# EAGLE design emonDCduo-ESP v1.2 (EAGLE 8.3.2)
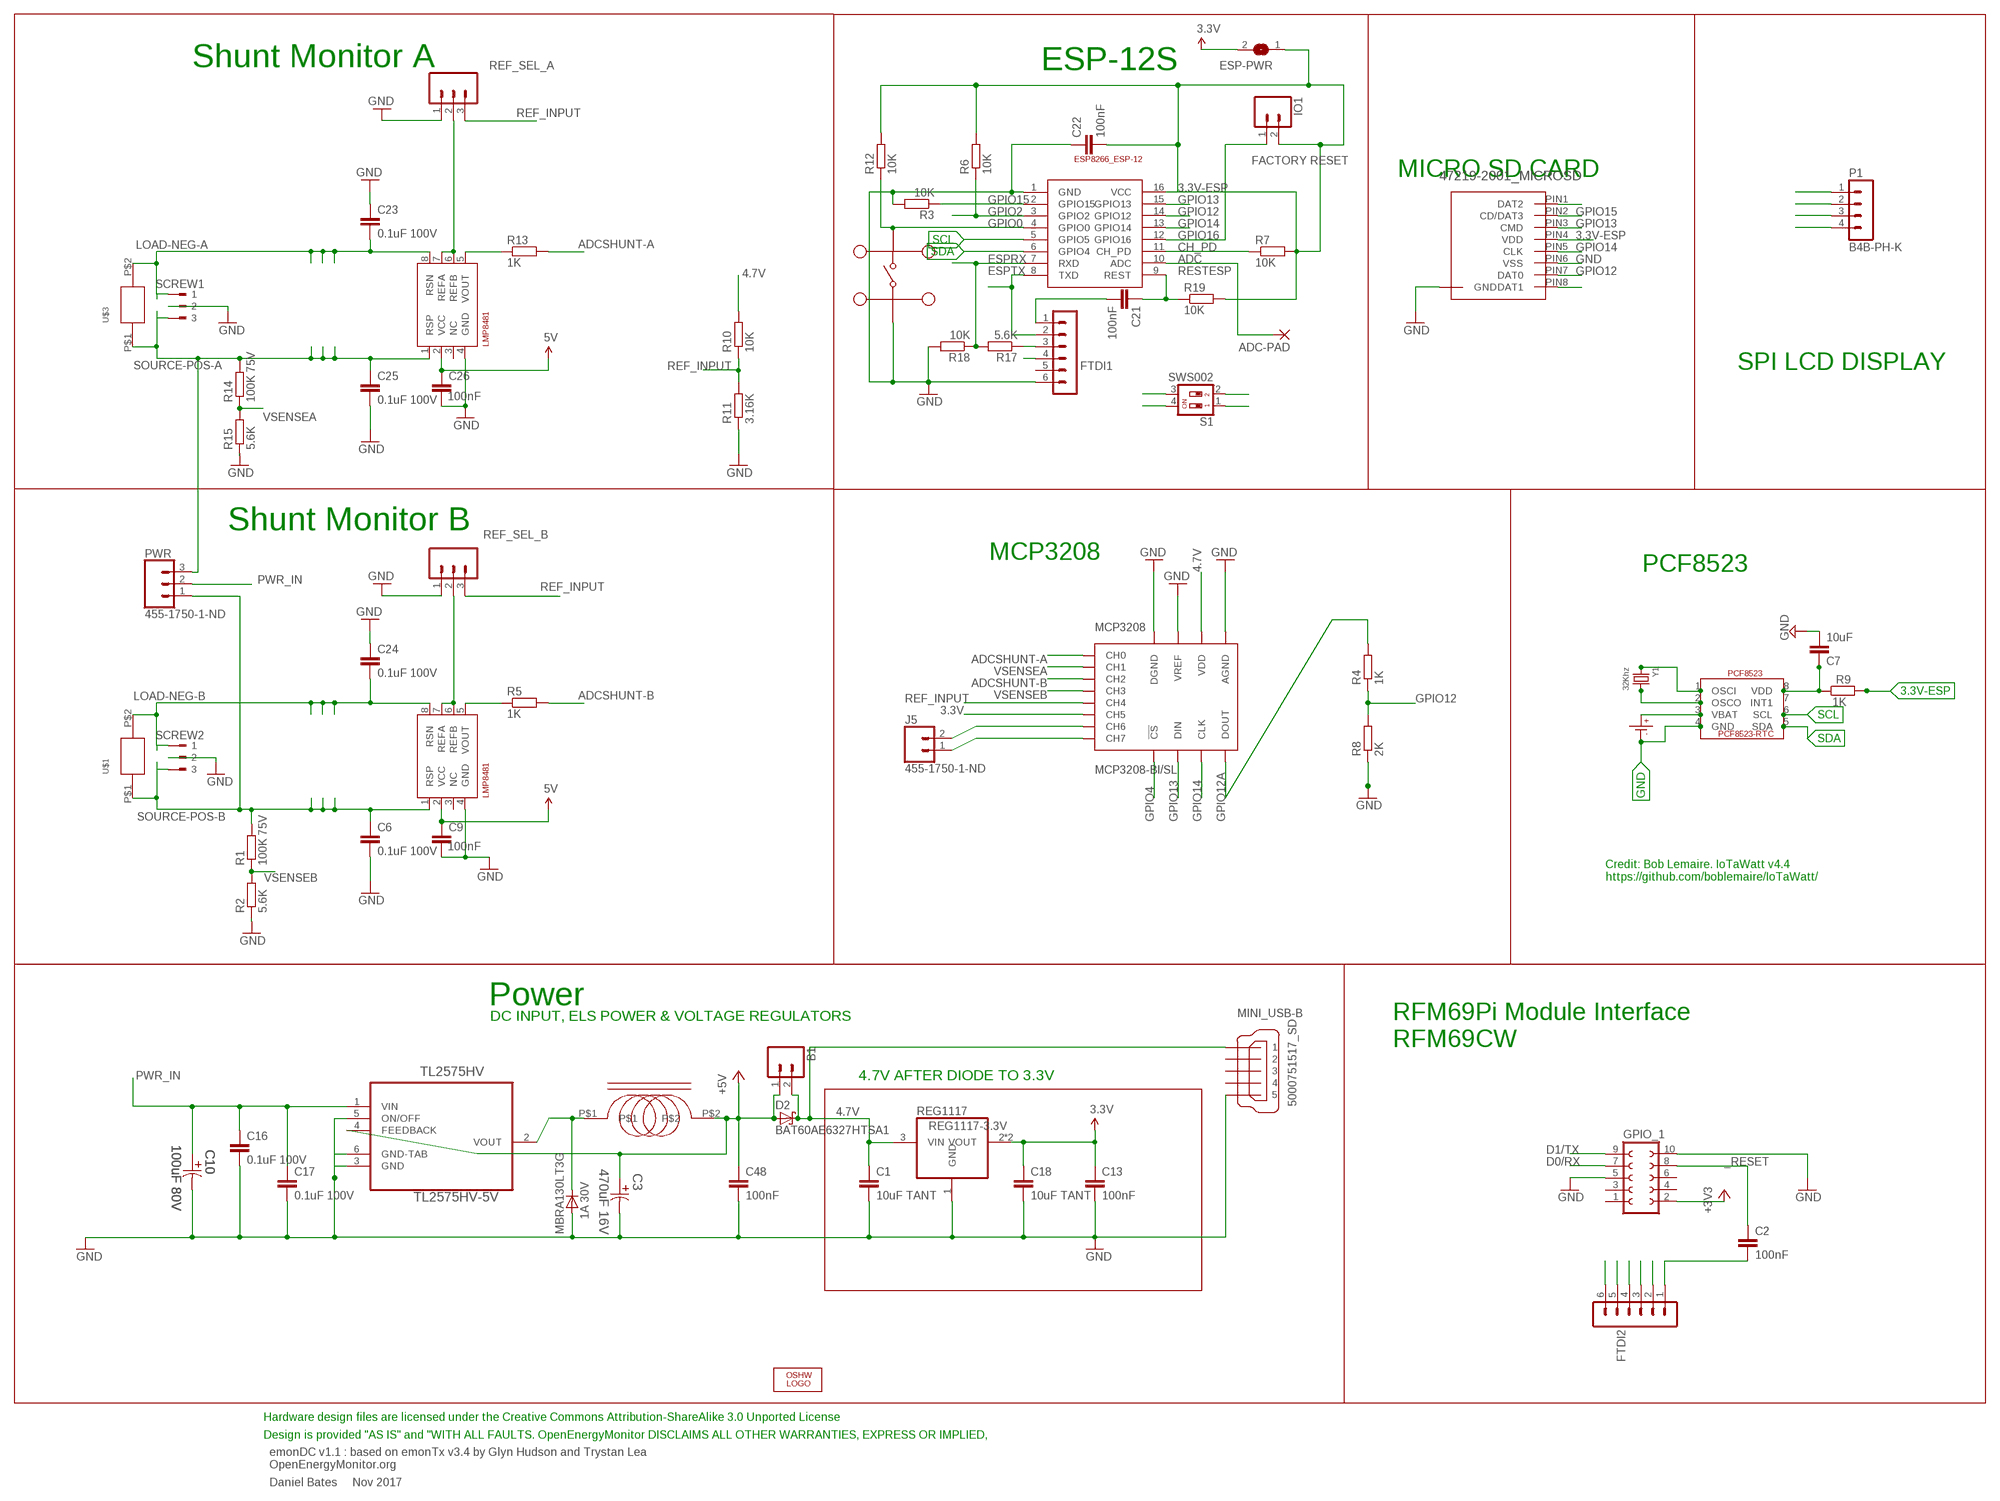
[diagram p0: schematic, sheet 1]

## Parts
ADC-PAD  2,15/1,0  [2,15/1,0]
B1  M02PTH  [1X02]
C1  10uF TANT  C-EUC0603  [C0603]
C2  100nF  C-EUC0603  [C0603]
C3  470uF 16V  EEE-FK1C471P-CASE-F  [CAPAE830X1050N]
C6  0.1uF 100V  C-EUC0603  [C0603]
C7  10uF  C-EUC0603  [C0603]
C9  100nF  C-EUC0603  [C0603]
C10  100uF 80V  EEV-FK1K101Q-CASE-H13  [CAPAE1350X1400N]
C13  100nF  C-EUC0603  [C0603]
C16  0.1uF 100V  C-EUC0603  [C0603]
C17  0.1uF 100V  C-EUC0603  [C0603]
C18  10uF TANT  C-EUC0603  [C0603]
C21  100nF  C-EUC0603  [C0603]
C22  100nF  C-EUC0603  [C0603]
C23  0.1uF 100V  C-EUC0603  [C0603]
C24  0.1uF 100V  C-EUC0603  [C0603]
C25  0.1uF 100V  C-EUC0603  [C0603]
C26  100nF  C-EUC0603  [C0603]
C48  100nF  C-EUC0603  [C0603]
CR1220  CR1220SMD  [CR1220SMD]
D1  MBRA130LT3G  [DO-214]
D2  BAT60AE6327HTSA1  BAT60J  [SOD323_ST]
ESP-12  ESP8266_ESP-12  [ESP8266-ESP12]
ESP-PWR  SJ  [SJ]
FTDI1  FTDI  MA06-1  [MA06-1]
FTDI2  FTDI  MA06-1  [MA06-1]
GPIO_1  FE05-2  [FE05-2]
I1  330uH  SRR0603-331KL  [SRR0603-331KL]
IO1  M02PTH  [1X02]
J5  455-1750-1-ND  CONN_02  [1X02]
LOGO1  OSHW_LOGO_6MILX0200-NT  [OSHW_6X200_NOTEXT]
MC2  MC32882  [SWITCH_TACT_MULTICOMP]
MCP3208  MCP3208-BI/SL  [SOIC16]
MINI_USB-B  5000751517_SD  [5000751517_SD]
P1  B4B-PH-K  [B4B-PH-K]
PCF8523  PCF8523_RTC  [SOIC_8]
PWR  455-1750-1-ND  CONN_03  [1X03]
R1  100K 75V  R-EU_R0603  [R0603]
R2  5.6K  R-EU_R0603  [R0603]
R3  10K  R-EU_R0603  [R0603]
R4  1K  R-EU_R0603  [R0603]
R5  1K  R-EU_R0603  [R0603]
R6  10K  R-EU_R0603  [R0603]
R7  10K  R-EU_R0603  [R0603]
R8  2K  R-EU_R0603  [R0603]
R9  1K  R-EU_R0603  [R0603]
R10  10K  R-EU_0309/12  [0309/12]
R11  3.16K  R-EU_0309/12  [0309/12]
R12  10K  R-EU_R0603  [R0603]
R13  1K  R-EU_R0603  [R0603]
R14  100K 75V  R-EU_R0603  [R0603]
R15  5.6K  R-EU_R0603  [R0603]
R17  5.6K  R-EU_R0603  [R0603]
R18  10K  R-EU_R0603  [R0603]
R19  10K  R-EU_R0603  [R0603]
REF_SEL_A  455-1750-1-ND  CONN_03  [1X03]
REF_SEL_B  455-1750-1-ND  CONN_03  [1X03]
REG1117  REG1117-3.3V  REG1117-VOUT4  [SOT223]
S1  SWS002  [SMS-002]
SCREW1  180-3  [180-3]
SCREW2  180-3  [180-3]
SHUNTMON-A  LMP8481  LMP8481-H  [S-PDSO-G08]
SHUNTMON-B  LMP8481  LMP8481-H  [S-PDSO-G08]
TL2575HV  TL2575HV-5V  TL2575HV-05IKTTR  [TO-263]
U$1  EBW_SERIES_15.2MM  [EBW_SERIES_15.2MM]
U$3  EBW_SERIES_15.2MM  [EBW_SERIES_15.2MM]
U$4  47219-2001_MICROSD  [47219-2001_MICROSD]
Y1  32Khz  CRYSTAL8X3.8SMT  [CRYSTAL_8X3.8]

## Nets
3.3V: C13.1 C18.1 ESP-PWR.2 GPIO_1.2 MCP3208.6(CH5) P1.3 REG1117.2(VOUT) REG1117.4(VOUT) ; supply symbol labelled +3V3
3.3V-ESP: C22.2 ESP-12.16(VCC) ESP-PWR.1 IO1.2 R6.2 R7.2 R9.2 R12.2 R19.2 U$4.PIN4(VDD)
4.7V [power]: B1.2 C1.1 C9.1 C26.1 D2.C FTDI1.4 FTDI2.4 MCP3208.16(VDD) MINI_USB-B.VBUS R10.2 REG1117.3(VIN) SHUNTMON-A.2(VCC) SHUNTMON-B.2(VCC) ; supply symbol labelled 5V
+5V: B1.1 C3.1 C48.1 D2.A I1.P$2 TL2575HV.4(FEEDBACK)
_RESET: C2.1 GPIO_1.8
ADC: ADC-PAD.1(P) ESP-12.10(ADC)
ADCSHUNT-A: MCP3208.1(CH0) R13.2
ADCSHUNT-B: MCP3208.3(CH2) R5.2
CH6: J5.2 MCP3208.7(CH6)
CH7: J5.1 MCP3208.8(CH7)
CH_PD: ESP-12.11(CH_PD) R7.1
D0/RX: FTDI2.2 GPIO_1.7 S1.2
D1/TX: FTDI2.3 GPIO_1.9 S1.1
ESPRX: ESP-12.7(RXD) R17.2 R18.1 S1.4
ESPTX: ESP-12.8(TXD) FTDI1.2 S1.3
GND [thin_power]: C1.2 C3.2 C6.2 C7.2 C9.2 C10.2 C13.2 C16.2 C17.2 C18.2 C22.1 C23.1 C24.1 C25.2 C26.2 C48.2 CR1220.P-(P$-) D1.P$2(A) ESP-12.1(GND) FTDI1.6 FTDI2.6 GPIO_1.5 GPIO_1.10 MC2.P$1 MC2.P$2 MCP3208.9(DGND) MCP3208.14(AGND) MCP3208.15(VREF) MINI_USB-B.GND1 MINI_USB-B.GND2 MINI_USB-B.GND3 P1.4 PCF8523.4(GND) R2.1 R3.2 R8.1 R11.1 R15.1 R18.2 REF_SEL_A.1 REF_SEL_B.1 REG1117.1(GND) SCREW1.2 SCREW2.2 SHUNTMON-A.4(GND) SHUNTMON-B.4(GND) TL2575HV.3(GND) TL2575HV.5(ON/OFF) TL2575HV.6(GND-TAB) U$4.P$1(GND) U$4.P$2(GND) U$4.P$3(GND) U$4.P$4(GND) U$4.PIN6(VSS)
GPIO0: ESP-12.4(GPIO0) MC2.P$3 MC2.P$4 R12.1
GPIO2: ESP-12.3(GPIO2) R6.1
GPIO4: MCP3208.10(!CS)
GPIO12: ESP-12.14(GPIO12) R4.1 R8.2 U$4.PIN7(DAT0)
GPIO12A: MCP3208.12(DOUT) R4.2
GPIO13: ESP-12.15(GPIO13) MCP3208.11(DIN) U$4.PIN3(CMD)
GPIO14: ESP-12.13(GPIO14) MCP3208.13(CLK) U$4.PIN5(CLK)
GPIO15 [thin_power]: ESP-12.2(GPIO15) R3.1 U$4.PIN2(CD/DAT3)
GPIO16: ESP-12.12(GPIO16) IO1.1
IND: D1.P$1(C) I1.P$1 TL2575HV.2(VOUT)
LOAD-NEG-A: C23.2 SCREW1.1 SHUNTMON-A.8(RSN) U$3.P$2
LOAD-NEG-B: C24.2 SCREW2.1 SHUNTMON-B.8(RSN) U$1.P$2
N$4: R13.1 SHUNTMON-A.5(VOUT)
N$6: R5.1 SHUNTMON-B.5(VOUT)
N$7: U$4.PIN1(DAT2)
N$10: C7.1 PCF8523.8(VDD) R9.1
N$20: FTDI2.5
N$30: C21.2 FTDI1.1
N$32: U$4.PIN8(DAT1)
N$36: FTDI1.3 R17.1
N$43: CR1220.P+(P$+) PCF8523.3(VBAT)
N$44: PCF8523.2(OSCO) Y1.P$4
N$45: PCF8523.1(OSCI) Y1.P$1
N$301: C2.2 FTDI2.1
PWR_IN: C10.1 C16.1 C17.1 PWR.2 TL2575HV.1(VIN)
REF_A_INPUT: REF_SEL_A.2 SHUNTMON-A.6(REFB) SHUNTMON-A.7(REFA)
REF_B_INPUT [thin_power]: REF_SEL_B.2 SHUNTMON-B.6(REFB) SHUNTMON-B.7(REFA)
REF_INPUT: MCP3208.5(CH4) R10.1 R11.2 REF_SEL_A.3 REF_SEL_B.3
RESTESP: C21.1 ESP-12.9(REST) R19.1
SCL: ESP-12.5(GPIO5) P1.2 PCF8523.6(SCL)
SDA: ESP-12.6(GPIO4) P1.1 PCF8523.5(SDA)
SOURCE-POS-A: C25.1 PWR.3 R14.2 SCREW1.3 SHUNTMON-A.1(RSP) U$3.P$1
SOURCE-POS-B: C6.1 PWR.1 R1.2 SCREW2.3 SHUNTMON-B.1(RSP) U$1.P$1
VSENSEA: MCP3208.2(CH1) R14.1 R15.2
VSENSEB: MCP3208.4(CH3) R1.1 R2.2
Unconnected: FTDI1.5 GPIO_1.1 GPIO_1.3 GPIO_1.4 GPIO_1.6 MINI_USB-B.D+ MINI_USB-B.D- MINI_USB-B.ID PCF8523.7(INT1) SHUNTMON-A.3(NC) SHUNTMON-B.3(NC)

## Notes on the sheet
- Shunt Monitor A | ESP-12S
- FACTORY RESET
- MICRO SD CARD
- SPI LCD DISPLAY
- Shunt Monitor B
- MCP3208
- PCF8523
- Credit: Bob Lemaire. IoTaWatt v4.4
  https://github.com/boblemaire/IoTaWatt/
- Power
- DC INPUT, ELS POWER & VOLTAGE REGULATORS
- RFM69Pi Module Interface
  RFM69CW
- 4.7V AFTER DIODE TO 3.3V
- Hardware design files are licensed under the Creative Commons Attribution-ShareAlike 3.0 Unported License
- Design is provided "AS IS" and "WITH ALL FAULTS. OpenEnergyMonitor DISCLAIMS ALL OTHER WARRANTIES, EXPRESS OR IMPLIED,
- emonDC v1.1 : based on emonTx v3.4 by Glyn Hudson and Trystan Lea
  OpenEnergyMonitor.org
- Daniel Bates     Nov 2017

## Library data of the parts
ADC-PAD = wirepad:2,15/1,0: THROUGH-HOLE PAD
B1 IO1 = SparkFun:M02: Header 2
C1 C2 C7 C13 C16-C18 C21 C22 C48 = rcl:C-EU: CAPACITOR, European symbol
C3 = Panasonic-EEEFK_EEEFP:EEE-: Aluminum Electrolytic Capacitors,Surface Mount Type; MPN: EEE-FK1C471P; OC_FARNELL: 9695710; OC_NEWARK: 96K9385; PACKAGE: CASE-F; SUPPLIER: PANASONIC; TOLERANCE: ±20 %; VALUE: 470UF; VOLTAGERATING: 16V
C6 C9 C23-C26 = rcl:C-EU: CAPACITOR, European symbol; MPN: C1608X7S2A104K080AB
C10 = Panasonic-EEE-EEV-EEF-ECQ:EEV-: Aluminum Electrolytic Capacitors,Surface Mount Type; MPN: EEVFK1K101Q; OC_FARNELL: 9696113; OC_NEWARK: 96K9484; SUPPLIER: PANASONIC; TOLERANCE: ±20 %; VALUE: 100UF; VOLTAGERATING: 80V
CR1220 = IotaWatt_parts:CR1220SMD: CR1220 Battery SMD
D1 = CASE 403D Diode:MBRA130LT3G: Fast switching diode; MF: ON SEMICONDUCTOR; MPN: MBRA130LT3G; OC_FARNELL: 9555978
D2 = diode:BAT60J: Schottky barrier diode
ESP-12 = ESP8266-ESP12:ESP8266_ESP-12
ESP-PWR = jumper:SJ: SMD solder JUMPER
FTDI1 FTDI2 = JeeLabs:MA06-1: PIN HEADER
GPIO_1 = con-lsta:FE05-2: FEMALE HEADER; OC_FARNELL: unknown; OC_NEWARK: unknown
I1 = SRR0603-331KL:SRR0603-331KL: SRR0603-331KL; INDUCTANCE: 330uH; MF: BOURNS; MPN: SRR0603-331KL; OC_FARNELL: 2333890
J5 = SparkFun-Connectors:CONN_02: Multi connection point. Often used as Generic Header-pin footprint for 0.1 inch spaced/style header connections
LOGO1 = ohw-logo:OSHW_LOGO_6MIL; OC_FARNELL: unknown
MC2 = multicomp tact switch:MC32882
MCP3208 = MCP3208:MCP3208
MINI_USB-B = 5000751517_sd:5000751517_SD
P1 = jst-ph:B4B-PH-K: HEADER
PCF8523 = IotaWatt_parts:PCF8523_RTC: PCF8523-RTC SOIC-8
PWR = SparkFun-Connectors:CONN_03: Multi connection point. Often used as Generic Header-pin footprint for 0.1 inch spaced/style header connections On any of the 0.1 inch spaced packages, you can populate with these: Break Away Headers - Straight (PRT-00116) Break Away Male Headers - Right Angle (PRT-00553) Female Headers (PRT-00115)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; PROD_ID: XXX-00000
R1 R14 = rcl:R-EU_: RESISTOR, European symbol; MPN: MCWR06X1003FTL
R2 R4 R8 R15 = rcl:R-EU_: RESISTOR, European symbol; MPN: MCWR06X5901FTL
R3 R5-R7 R9-R13 R17-R19 = rcl:R-EU_: RESISTOR, European symbol
REF_SEL_A REF_SEL_B = SparkFun-Connectors:CONN_03: Multi connection point. Often used as Generic Header-pin footprint for 0.1 inch spaced/style header connections On any of the 0.1 inch spaced packages, you can populate with these: Break Away Headers - Straight (PRT-00116) Break Away Male Headers - Right Angle (PRT-00553) Female Headers (PRT-00115)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; MF: MULTICOMP; MPN: 2212S-02SG-85; OC_FARNELL: 1593458; PROD_ID: XXX-00000
REG1117 = burr-brown:REG1117-VOUT4: 800mA and 1A Low Dropout (LDO) Positive Regulator 1.8V, 2.5V, 2.85V, 3.3V, 5V, and Adj; MF: TEXAS INSTRUMENTS; MPN: REG1117; OC_FARNELL: 1097566; OC_NEWARK: 14P6981
S1 = smd-special:SWS002: SMD Dip Switch 2 pol.
SCREW1 SCREW2 = con-weidmueller-sl35:180-3: WEIDMUELLER CLAMP CONNECTOR; OC_FARNELL: unknown; OC_NEWARK: unknown
SHUNTMON-A = lmp8481b:LMP8481: LMP8481MM-H/NOPB 100V/V; MF: TEXAS INSTRUMENTS; MPN: LMP8481MME-S/NOPB; OC_FARNELL: 2322044
SHUNTMON-B = lmp8481b:LMP8481: LMP8481MM-H/NOPB 100V/V; MF: TEXAS INSTRUMENTS; MPN: LMP8481MME-H/NOPB; OC_FARNELL: 2322044
TL2575HV = TL2575HV:TL2575HV; MF: TEXAS INSTRUMENTS; MPN: LM2575HVS-15/NOPB; OC_FARNELL: 2492609
U$1 U$3 = EBW series shunt:EBW_SERIES_15.2MM
U$4 = MOLEX 47219-2001:47219-2001_MICROSD
Y1 = microbuilder:CRYSTAL: Crystals

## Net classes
2 thin_power: width 0.254 mm

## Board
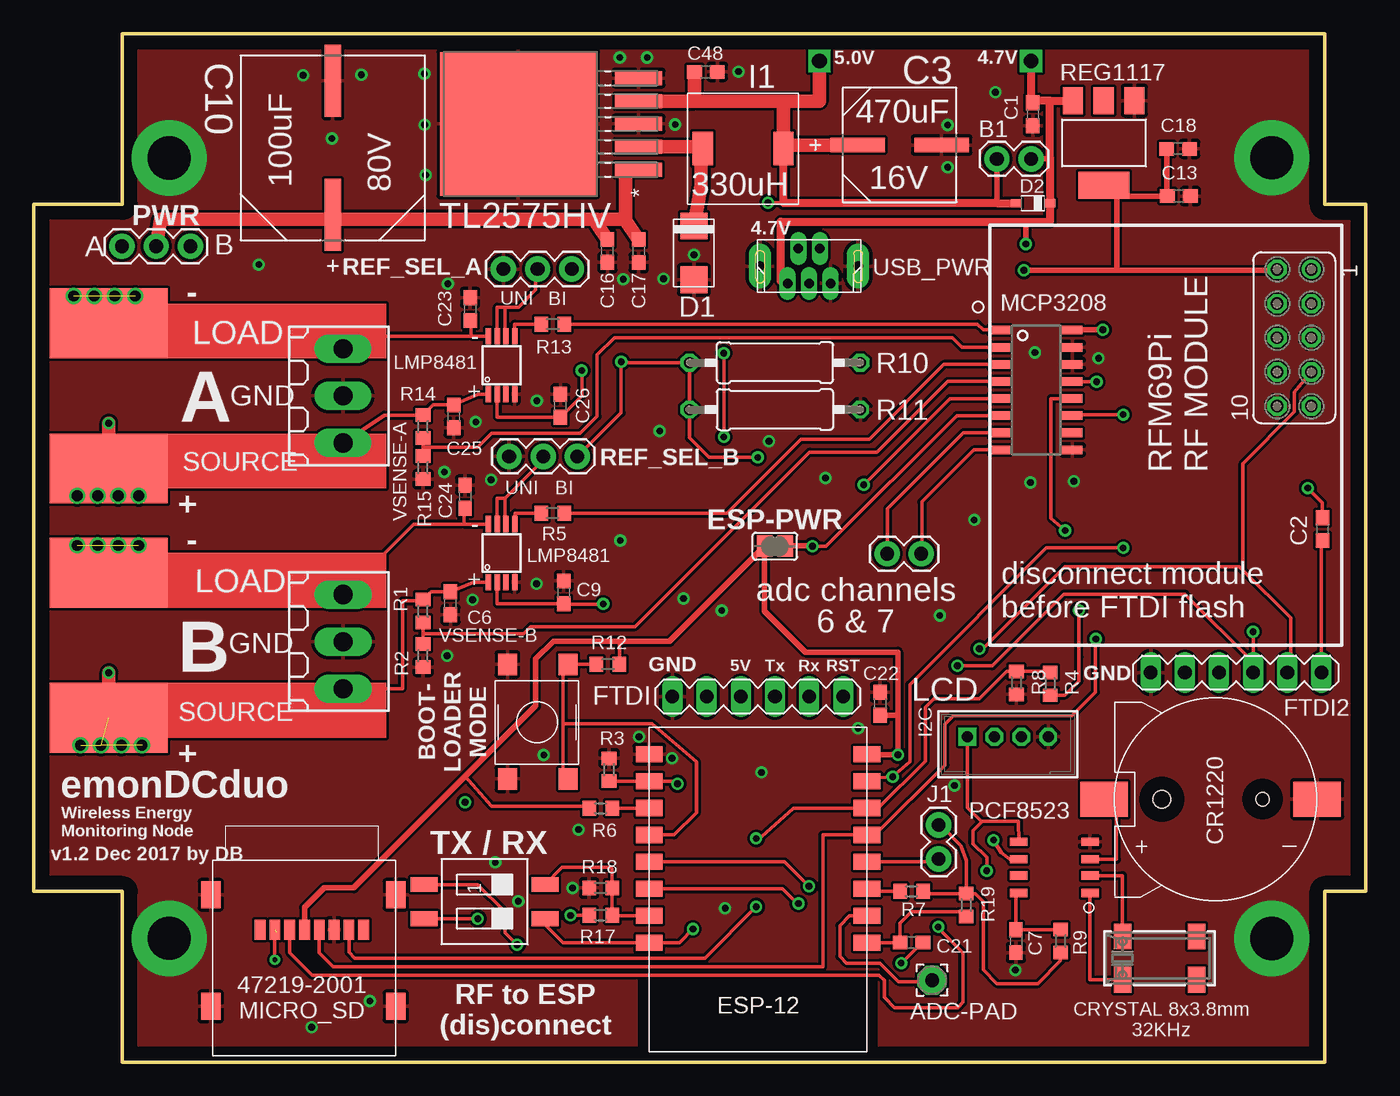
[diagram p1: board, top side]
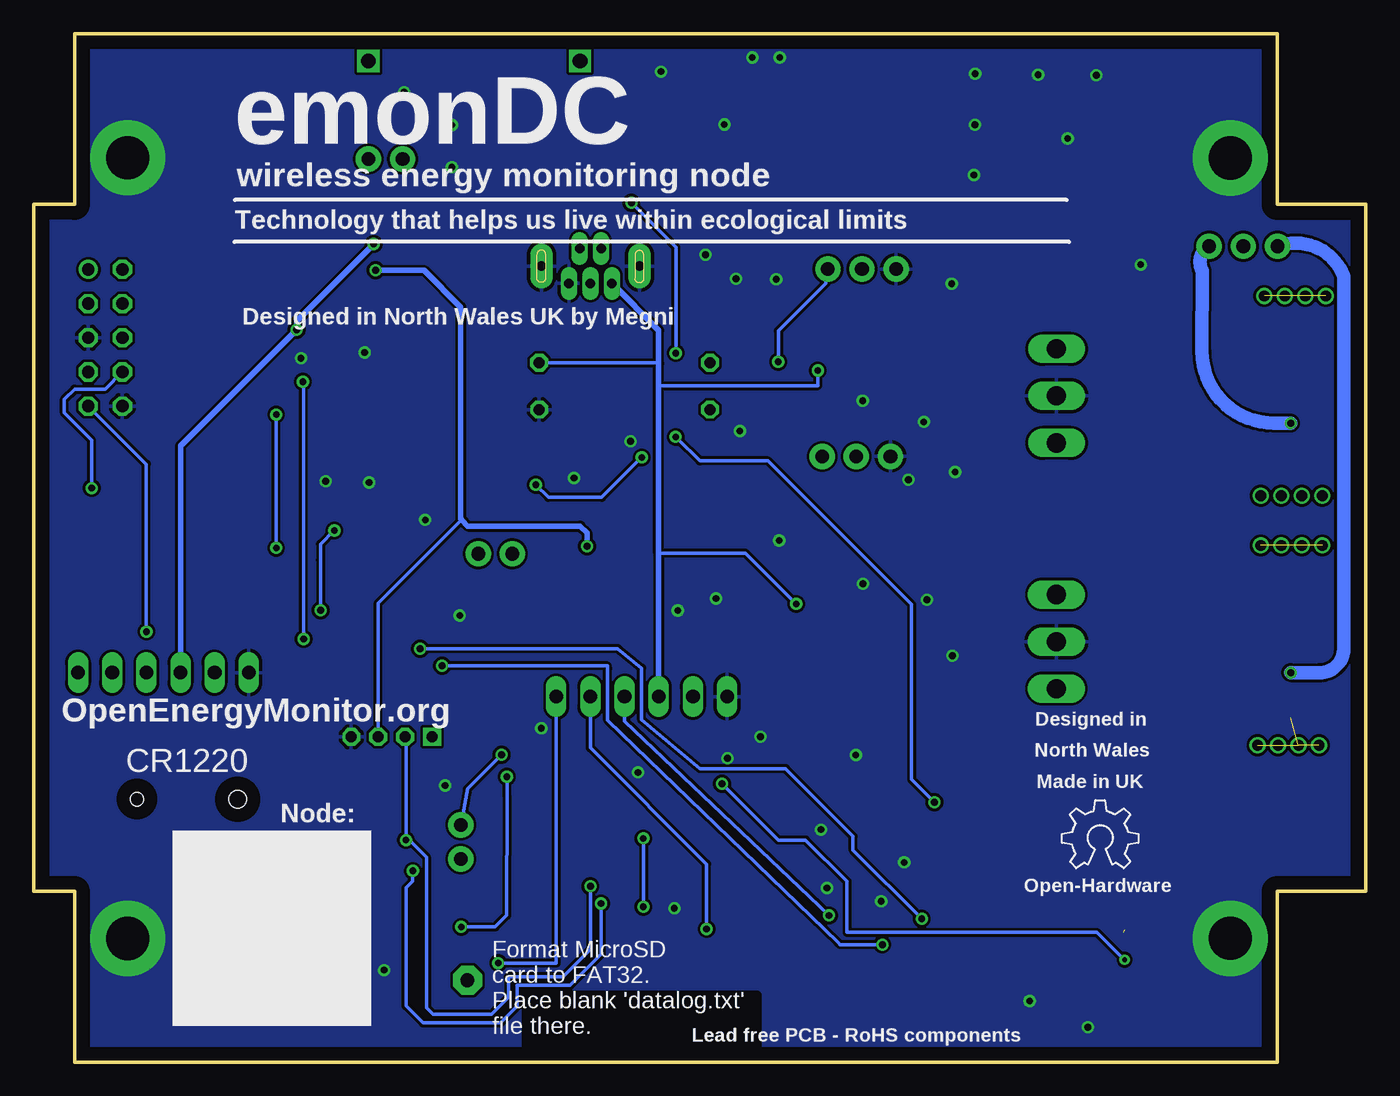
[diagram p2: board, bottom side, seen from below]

Size 99.06 x 76.45 mm. Coordinates in mm from the lower left corner, seen from the top.
Outline: 6.6,63.75 6.6,76.45 96.01,76.45 96.01,63.75 99.06,63.75 99.06,12.7 96.01,12.7 96.01,0 6.6,0 6.6,12.7 0,12.7 0,63.75 6.6,63.75
Copper layers (1*16): Top 0.035mm / dielectric 1.5mm / Bottom 0.035mm
Design rules "default *": minimum track width 10mil, minimum drill 19mil, track to track 8mil, track to pad 8mil, pad to pad 8mil, via to via 8mil, smd to smd 8mil, copper to edge 40mil, drill to drill 8mil, minimum pad ring 10mil, minimum via ring 8mil, stop-mask expansion 4mil, vias tented up to drill 0mil, thermal gap 10mil
tRestrict: area 45.2,1 to 62.5,6.1
bRestrict: area 45.2,1 to 62.5,5.1

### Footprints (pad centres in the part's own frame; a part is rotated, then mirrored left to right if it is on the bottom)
2,15/1,0 = drill 1.016 pad 2.159 octagon: 1 0,0
1X02 = drill 1.016 pad 1.88: 1 0,0; 2 2.54,0
C0603 = smd 1.1 x 1: 1 -0.85,0; 2 0.85,0
CAPAE830X1050N = smd 4.064 x 1.092: 1 -3.124,0; 2 3.124,0
CAPAE1350X1400N = smd 5.359 x 1.194: 1 -4.978,0; 2 4.978,0
CR1220SMD = smd 3.54 x 2.6: P+ 8.3,0; P- -7.55,0 | hole 1: -3.5,0 | hole 1.3: 4,0
DO-214 = smd 2 x 2: P$1 -2,0; P$2 2,0
SOD323_ST = smd 0.8 x 0.6: A 1.25,0; C -1.25,0
ESP8266-ESP12 = smd 2 x 1.2: 1 16.2,2; 2 16.2,4; 3 16.2,6; 4 16.2,8; 5 16.2,10; 6 16.2,12; 7 16.2,14; 8 16.2,16; 9 0,16; 10 0,14; 11 0,12; 12 0,10; 13 0,8; 14 0,6; 15 0,4; 16 0,2
SJ = smd 1.168 x 1.6: 1 -0.762,0; 2 0.762,0
MA06-1 = drill 1.016 long: 1 0,0; 2 2.54,0; 3 5.08,0; 4 7.62,0; 5 10.16,0; 6 12.7,0
FE05-2 = drill 0.914: 1 -5.08,1.27 | drill 0.914 octagon: 2 -5.08,-1.27; 3 -2.54,1.27; 4 -2.54,-1.27; 5 0,1.27; 6 0,-1.27; 7 2.54,1.27; 8 2.54,-1.27; 9 5.08,1.27; 10 5.08,-1.27
SRR0603-331KL = smd 1.5 x 2.5: P$1 -3,0; P$2 3,0
SWITCH_TACT_MULTICOMP = smd 1.6 x 1.4: P$1 -1.1,5.3; P$2 7.4,5.3; P$3 -1.1,0.8; P$4 7.4,0.8
SOIC16 = smd 0.635 x 1.524: 1 -4.445,-2.695; 2 -3.175,-2.695; 3 -1.905,-2.695; 4 -0.635,-2.695; 5 0.635,-2.695; 6 1.905,-2.695; 7 3.175,-2.695; 8 4.445,-2.695; 9 4.445,2.695; 10 3.175,2.695; 11 1.905,2.695; 12 0.635,2.695; 13 -0.635,2.695; 14 -1.905,2.695; 15 -3.175,2.695; 16 -4.445,2.695
5000751517_SD = drill 0.7 pad 1.016 long: D+ 0,-1.3; D- -0.8,1.3; GND1 1.6,-1.3; ID 0.8,1.3; VBUS -1.6,-1.3 | drill 0.7 pad 1.676 long: GND2 3.65,0; GND3 -3.65,0
B4B-PH-K = drill 0.813 square: 1 -3,0 | drill 0.813 octagon: 2 -1,0; 3 1,0; 4 3,0
SOIC_8 = smd 1.3 x 0.6: 1 -2.6,1.9; 2 -2.6,0.6; 3 -2.6,-0.6; 4 -2.6,-1.9; 5 2.7,-1.9; 6 2.7,-0.6; 7 2.7,0.6; 8 2.7,1.9
1X03 = drill 1.016 pad 1.88: 1 0,0; 2 2.54,0; 3 5.08,0
R0603 = smd 1 x 1.1: 1 -0.85,0; 2 0.85,0
0309/12 = drill 0.813 octagon: 1 -6.35,0; 2 6.35,0
SOT223 = smd 1.499 x 2.007: 1 -2.261,-3.15; 2 0.025,-3.15; 3 2.311,-3.15 | smd 3.81 x 2.007: 4 0,3.15
SMS-002 = smd 1.092 x 2.007: 1 -1.27,-4.496; 2 1.27,-4.496; 3 1.27,4.496; 4 -1.27,4.496
180-3 = drill 1.422 long: 1 -3.5,0; 2 0,0; 3 3.5,0
S-PDSO-G08 = smd 0.4 x 1.2: 1 -0.975,-2.157; 2 -0.325,-2.157; 3 0.325,-2.157; 4 0.975,-2.157; 5 0.975,2.157; 6 0.325,2.157; 7 -0.325,2.157; 8 -0.975,2.157
TO-263 = smd 1.041 x 3.505: 1 -3.404,-8.788; 2 -1.702,-8.788; 3 0,-8.788; 4 1.702,-8.788; 5 3.404,-8.788 | smd 10.668 x 11.659: 6 0,0.152
EBW_SERIES_15.2MM = smd 5.2 x 8.75: P$1 -5.4,0; P$2 5.4,0
47219-2001_MICROSD = smd 1.45 x 2: P$1 0,0; P$2 13.75,0; P$3 0,8.3; P$4 13.75,8.3 | smd 0.8 x 1.5: PIN1 10.08,2.6; PIN2 8.98,2.6; PIN3 7.88,2.6; PIN4 6.78,2.6; PIN5 5.68,2.6; PIN6 4.58,2.6; PIN7 3.48,2.6; PIN8 2.38,2.6
CRYSTAL_8X3.8 = smd 1.3 x 1.9: P$1 -2.75,-1.6; P$2 2.75,-1.6; P$3 2.75,1.6; P$4 -2.75,1.6

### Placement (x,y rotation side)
ADC-PAD  66.8,6.1 0 top
B1  71.63,67.14 0 top
C1  74.3,70.46 270 top
C2  95.83,39.63 270 top
C3  64.39,68.17 0 top
C6  30.99,34.11 270 top
C7  73.04,9 270 top
C9  39.42,34.93 90 top
C10  22.25,67.96 90 top
C13  85.15,64.38 0 top
C16  42.66,60.3 270 top
C17  44.99,60.3 270 top
C18  85.1,67.89 0 top
C21  65.28,8.89 0 top
C22  62.94,26.64 270 top
C23  32.46,55.98 270 top
C24  32.08,42.04 270 top
C25  31.24,48.01 270 top
C26  39.17,48.8 90 top
C48  49.99,73.61 0 top
CR1220  87.88,19.56 180 top
D1  49.09,60.16 270 top
D2  74.31,63.85 180 top
ESP-12  61.98,24.89 180 top
ESP-PWR  55.12,38.35 0 top
FTDI1  60.2,27.18 180 top
FTDI2  95.76,28.96 180 top
GPIO_1  93.73,53.85 270 top
I1  52.76,67.91 0 top
IO1  67.29,15.1 90 top
J5  66,37.79 180 top
LOGO1  22.6,14.4 0 bottom
MC2  40.53,22.17 90 top
MCP3208  74.54,49.96 270 top
MINI_USB-B  57.66,59.18 0 top
P1  72.44,24.18 0 top
PCF8523  75.95,14.48 180 top
PWR  6.57,60.64 0 top
R1  28.96,33.53 90 top
R2  28.96,30.23 90 top
R3  42.79,21.74 90 top
R4  75.57,28.13 270 top
R5  38.6,40.81 0 top
R6  42.16,18.87 180 top
R7  65.28,12.7 0 top
R8  73.08,28.19 90 top
R9  76.36,9.01 270 top
R10  55.12,52 0 top
R11  55.12,48.51 180 top
R12  42.7,29.59 0 top
R13  38.61,54.86 0 top
R14  28.96,47.24 90 top
R15  28.96,44.2 90 top
R17  42.16,10.92 0 top
R18  42.16,12.95 180 top
R19  69.34,11.68 90 top
REF_SEL_A  34.92,58.95 0 top
REF_SEL_B  35.35,45.03 0 top
REG1117  79.58,68.33 180 top
S1  33.53,11.94 270 top
SCREW1  23,49.53 270 top
SCREW2  23.01,31.26 270 top
SHUNTMON-A  34.8,51.82 0 top
SHUNTMON-B  34.8,37.85 0 top
TL2575HV  36.19,69.74 90 top
U$1  5.59,30.99 90 top
U$3  5.59,49.53 90 top
U$4  26.92,12.45 180 top
Y1  83.71,7.73 0 top

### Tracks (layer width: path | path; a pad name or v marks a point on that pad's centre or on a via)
3.3V  (via drill 0.5)
  Top 0.254: 55.94,38.39 ESP-PWR.2 | 92.46,58.86 GPIO_1.2 | MCP3208.6 68.63,48.06 58.93,38.35 v57.91,38.35
  Top 0.406: REG1117.2 79.54,71.48 | C18.1 84.25,64.44 C13.1 80.55,64.38 | 79.54,65.13 REG1117.4 79.58,64.38 80.55,64.38 | v57.91,38.35 57.88,38.39 55.94,38.39 | v73.63,58.86 80.55,58.86 | 80.55,58.86 92.46,58.86 | 80.55,58.86 80.55,64.38
  Bottom 0.254: P1.3 73.44,34.13 67.25,40.32
  Bottom 0.406: v73.63,58.86 70.04,58.86 67.31,56.13 67.31,40.39 67.25,40.32 66.78,39.85 58.42,39.85 57.91,39.34 v57.91,38.35
3.3V-ESP  (via drill 0.5)
  Top 0.254: R7.2 66.13,12.53 R19.2 | R6.2 40.89,19.04 34.05,19.04 32.09,21.25 | R19.2 69.34,14.99 68.96,16.11 67.42,17.64 IO1.2 | R19.2 70.02,12.53 70.61,11.94 70.61,6.86 71.63,5.84 74.68,5.84 76.36,7.53 R9.2 | R12.2 43.55,31.28 43.75,31.28
  Top 0.406: 64.26,25.91 64.26,30.48 57.4,30.48 54.36,33.53 ESP-PWR.1 47.29,31.28 43.75,31.28 38.65,31.28 37.34,29.97 37.34,26.49 32.09,21.25 23.8,12.95 21.59,12.95 20.14,11.51 U$4.PIN4 | 64.26,25.91 v64.26,22.86 62.01,22.86 ESP-12.16 | C22.2 64.15,25.8 64.26,25.91
  Bottom 0.254: v64.26,22.86 66.8,20.32 IO1.2
4.7V  (via drill 0.5, 1.1)
  Top 0.254: SHUNTMON-A.2 34.47,47.95 C26.1 40.76,49.54 40.76,51.36 40.75,51.36 v40.75,51.41 | SHUNTMON-B.2 34.47,34.08 C9.1 39.46,34.04 42.42,34.04 42.39,34.07 v42.36,34.07
  Top 0.406: D2.C 75.74,64.1 | 74.17,71.31 C1.1 74.3,71.48 | 75.56,62.48 73.79,62.48 v73.79,60.81 | v79.5,54.44 77.27,54.44 MCP3208.16 | MINI_USB-B.VBUS 55.86,58.08 55.56,58.08 | B1.2 75.4,67.14 75.56,67.31
  Top 0.61: v74.17,74.42 74.17,71.31 | 75.56,71.48 75.56,67.31 D2.C 75.56,62.48 55.56,62.48 55.56,58.08 | 75.56,71.48 REG1117.3 | 75.56,71.48 74.3,71.48
  Bottom 0.254: 40.85,51.31 v40.75,51.41 40.75,50.29 52.58,50.29 52.58,51.94 52.58,52 R10.2 | v42.36,34.07 46.14,37.85 52.58,37.85
  Bottom 0.406: FTDI1.4 52.58,37.85 52.58,51.94 52.58,54.4 MINI_USB-B.VBUS | FTDI2.4 88.14,45.81 v79.5,54.44 79.5,55.09 v73.79,60.81
+5V  (via drill 0.5, 1.1)
  Top 0.254: v54.61,63.88 55.72,63.88 55.76,63.85 | 32.07,19.16 v32.08,19.33 | v51.32,46.48 51.32,52.69 v51.31,52.7
  Top 0.406: B1.1 71.63,63.85
  Top 0.61: D2.A 71.63,63.85 55.76,63.85 I1.P$2
  Top 1.016: TL2575HV.4 49.14,71.44 | 49.14,71.44 C48.1 | 55.76,71.44 I1.P$2 55.5,68.17 C3.1 | 55.76,71.44 49.14,71.44 | v58.42,74.42 58.42,71.44 55.76,71.44
  Bottom 0.254: v51.32,46.48 51.18,46.36 49.53,44.7 44.45,44.7 33.78,34.04 33.78,21.03 v32.08,19.33 | v51.31,52.7 51.31,60.58 v54.61,63.88
_RESET  (via drill 0.5)
  Top 0.254: C2.1 95.83,41.58 v94.74,42.67
  Bottom 0.254: v94.74,42.67 94.74,46.23 96.77,48.26 96.77,49.28 96.01,50.04 93.73,50.04 GPIO_1.8
ADC
  Top 0.254: ESP-12.10 60.68,10.89 59.94,10.16 59.94,7.87 60.45,7.37 62.93,7.37 64.3,5.99 66.7,5.99 ADC-PAD.1
ADCSHUNT-A
  Top 0.254: R13.2 70.18,54.86 70.6,54.44 71.81,54.44 MCP3208.1
ADCSHUNT-B
  Top 0.254: MCP3208.3 71.82,51.88 67.69,51.88 62.14,46.32 57.05,46.32 51.54,40.81 R5.2 39.43,40.83
CH6
  Top 0.254: MCP3208.7 69.14,46.79 63.5,41.15 63.5,37.39 J5.2
CH7
  Top 0.254: MCP3208.8 69.9,45.52 66.04,41.66 66.04,37.39 J5.1
CH_PD
  Top 0.254: ESP-12.11 61.98,12.7 R7.1
D0/RX  (via drill 0.5)
  Top 0.254: S1.2 v33.02,10.67 | v70.32,30.73 70.57,30.73 76.67,36.83 89.66,36.83 89.92,36.58 | 89.92,36.58 93.47,33.02 93.47,29.21 FTDI2.2 | GPIO_1.7 93.75,49.81 93.75,48.34 89.92,44.5 89.92,36.58
  Bottom 0.254: v33.02,10.67 38.13,15.77 38.13,16.79 43.16,21.82 49.52,21.82 53.86,25.46 53.86,29.29 55.63,30.73 v70.32,30.73
D1/TX  (via drill 0.5)
  Top 0.254: v90.68,32 FTDI2.3 90.68,29.72 85.6,34.8 76.62,34.8 71.28,29.46 v68.69,29.46 | v35.95,8.74 35.05,9.64 35.05,11.18 33.02,13.21 S1.1
  Bottom 0.254: v68.69,29.46 56.39,29.46 56.38,29.26 56.38,25.43 39.22,8.87 39.1,8.74 v35.95,8.74 | v90.68,32 90.68,44.45 GPIO_1.9
ESPRX
  Top 0.254: ESP-12.7 42.79,10.89 R17.2 R18.1 43.01,14.39 42.93,14.48 39.29,14.48 S1.4
ESPTX  (via drill 0.5)
  Top 0.254: S1.3 38.02,10.24 39.37,8.89 ESP-12.8 48.01,8.89 v49.02,9.91
  Bottom 0.254: v49.02,9.91 49.02,14.73 57.66,23.37 FTDI1.2
GND  (via drill 0.5, 3.2 pad 5.59)
  Top 0.254: ESP-12.1 46.06,22.61
  other vias: 10.08,67.21 92.07,67.23 52.4,73.63 10.08,9.2 92.07,9.2 32.65,34.38 16.74,59.28 30.55,43.87 37.41,49.17 71.51,72.1 32.87,47.6 37.39,35.57 47.47,22.6 51.42,11.44 43.84,58.2 67.97,66.53 47.7,69.7 29.07,69.69 20.04,73.36 24.38,73.4 30.74,30.22 34.01,43.3 20.66,2.6 49.09,60.02 45.02,24.2 61.31,24.82 30.81,57.87 37.93,22.83 25.01,4.55 46.83,58.24 67.97,69.67 29.14,65.95 29.06,73.48 43.59,74.69 45.62,74.69 22.18,68.66 43.63,38.79 48.33,34.47 51.17,33.58 67.38,33.2 54.12,21.54 74.11,43.09 79.18,52.33 74.44,52.76 77.35,43.18 54.68,46.15 72.99,6.85 46.55,46.91 58.88,43.42 40.08,12.95 40.52,17.29 36.04,11.96 34.32,14.85 69.94,40.31 68.47,20.57
  pour Bottom (isolate 0.127): 6.86,76.2 6.86,63.5 0.25,63.5 0.25,12.95 6.86,12.95 6.86,0.25 95.76,0.25 95.76,12.95 98.81,12.95 98.81,63.5 95.76,63.5 95.76,76.2
  pour Top (isolate 0.127): 6.86,76.2 6.86,63.5 0.25,63.5 0.25,12.95 6.86,12.95 6.86,0.25 95.76,0.25 95.76,12.95 98.81,12.95 98.81,63.5 95.76,63.5 95.76,76.2
GPIO0
  Top 0.254: ESP-12.4 47.63,16.89 49.28,18.54 49.28,22.35 45.97,25.15 39.37,25.15 | 39.37,25.15 39.37,29.21 39.73,29.21 MC2.P$4 R12.1 | 39.37,25.15 39.37,21.59 39.73,21.59 MC2.P$3
GPIO2
  Top 0.254: 42.93,18.78 R6.1 45.76,18.87 ESP-12.3
GPIO12  (via drill 0.5)
  Top 0.254: 53.78,16.45 56.48,18.89 ESP-12.14 61.98,18.86 62.77,18.86 66.29,22.38 66.29,26.37 66.95,27.02 70.33,27.02 72.35,29.04 R8.2 75.57,29.04 R4.1 | 53.78,16.45 53.59,16.51 | v53.72,11.56 49.91,7.75 23.88,7.75 23.44,8.18 U$4.PIN7 | v53.72,16.64 53.85,16.64 53.78,16.45
  Bottom 0.254: v53.72,16.64 v53.72,11.56
GPIO12A  (via drill 0.5)
  Top 0.254: 77.22,49.34 MCP3208.12 75.64,49.33 75.64,40.45 76.69,39.52 v76.7,39.52 | v77.72,33.59 77.72,30.14 77.72,30.13 77.72,28.32 76.68,27.28 R4.2
  Bottom 0.254: v76.7,39.52 77.72,38.5 77.72,37.34 v77.72,33.59
GPIO13  (via drill 0.48, 0.5)
  Top 0.254: ESP-12.15 61.98,21.08 v63.87,21.22 65.15,22.35 65.15,28.07 75.31,38.23 v81.03,38.23 | v81.03,48.13 77.72,48.13 MCP3208.11 | v67.26,10.06 67.26,9.95 69.09,8.13 69.09,4.45 68.71,4.06 64.01,4.06 63.25,4.83 63.25,6.1 62.87,6.48 20.7,6.48 19.04,8.13 U$4.PIN3
  Bottom 0.254: v63.87,21.22 63.87,19.81 63.88,10.92 64.75,10.06 v67.26,10.06 | v81.03,38.23 v81.03,48.13
GPIO14  (via drill 0.5)
  Top 0.254: ESP-12.13 58.67,16.89 58.67,7.11 22.26,7.11 21.24,8.13 U$4.PIN5 | ESP-12.13 | ESP-12.13 62.57,16.89 67.77,22.08 67.77,25.14 68.38,25.76 77.19,25.76 78.95,27.52 78.95,31.43 v78.98,31.46 | v79.04,50.58 77.26,50.58 MCP3208.13
  Bottom 0.254: v78.98,31.46 78.98,50.52 v79.04,50.58
GPIO15  (via drill 0.35, 0.5)  (1 unrouted)
  Top 0.254: ESP-12.2 R3.1 47.88,20.89 v47.88,20.7 | 18.03,9.65 18.09,9.65 | v17.94,7.62 U$4.PIN2
  Bottom 0.254: v47.88,20.7 43.69,16.51 41.66,16.51 38.58,13.44 38.58,9.65 20,9.65 17.95,7.6 v17.94,7.62
GPIO16
  Top 0.254: IO1.1 66.71,14.89 ESP-12.12
IND
  Top 1.016: TL2575HV.2 49.63,68.04 | 49.63,68.04 I1.P$1 | 49.63,68.04 49.63,65.1 D1.P$1
LOAD-NEG-A
  Top 0.254: 32.51,53.97 23.94,53.97 SCREW1.1 22.34,53.69 7.02,53.69 | 32.51,53.97 SHUNTMON-A.8 | C23.2 32.51,54.83 32.51,53.97
  Top 2.54: 7.02,53.69 U$3.P$2
LOAD-NEG-B
  Top 0.152: U$1.P$2 5.59,37.85 5.6,37.86 | 8.69,38.35 8.69,38.05 7.03,36.39 U$1.P$2 | U$1.P$2 5.59,37.59 5.39,37.79 | U$1.P$2 5.91,36.39 7.25,37.73
  Top 0.254: 32,40 28.25,40 SCREW2.1 21.38,36.39 U$1.P$2 | 32,40 SHUNTMON-B.8 | C24.2 32,41.11 32,40
N$4
  Top 0.254: SHUNTMON-A.5 35.77,54.86 R13.1
N$6
  Top 0.254: SHUNTMON-B.5 35.81,40.81 R5.1
N$10
  Top 0.254: R9.1 73.05,9.86 C7.1 73.04,12.53 PCF8523.8
N$30  (via drill 0.5)
  Top 0.254: v64.52,7.37 66.04,8.89 C21.2
  Bottom 0.254: FTDI1.1 60.2,7.37 v64.52,7.37
N$36  (via drill 0.5)
  Top 0.254: R17.1 v39.92,10.91
  Bottom 0.254: v39.92,10.91 55.12,25.36 FTDI1.3
N$43
  Top 0.254: PCF8523.3 80.52,15.08 80.52,19.3 79.58,19.3 CR1220.P+
N$44
  Top 0.254: PCF8523.2 80.96,13.88 Y1.P$4
N$45
  Top 0.254: PCF8523.1 78.55,6.13 Y1.P$1
N$301
  Top 0.254: FTDI2.1 95.76,38.35 95.83,38.43 C2.2
PWR_IN
  Top 1.016: 44.27,66.33 TL2575HV.1 44.01,66.33 44.01,62.66 43.94,62.66 | PWR.2 9.46,62.66 21.93,62.66 | 43.94,62.66 42.29,62.66 41.9,62.27 | C16.1 41.9,62.27 | C17.1 43.97,62.63 43.94,62.66 | 21.93,62.66 C10.1 | 41.9,62.27 41.9,62.66 21.93,62.66
REF_A_INPUT
  Top 0.254: 35.05,56.13 35.05,54.04 SHUNTMON-A.6 | SHUNTMON-A.7 34.47,56.13 35.05,56.13 | 35.05,56.13 36.07,56.13 37.34,57.4 37.34,58.83 REF_SEL_A.2
REF_B_INPUT
  Top 0.254: REF_SEL_B.2 37.93,44.79 35.05,41.91 | 35.05,41.91 35.05,40.07 SHUNTMON-B.6 | SHUNTMON-B.7 34.47,41.91 35.05,41.91
REF_INPUT  (via drill 0.5)
  Top 0.254: v43.69,52.07 43.69,48.26 40.46,45.03 REF_SEL_B.3 | 43.69,52.32 v43.69,52.07 | v43.69,52.07 44.01,52.07 44.01,52 R10.1 R11.2 48.77,46.4 50.21,44.96 v53.85,44.96 | MCP3208.5 68.12,49.33 v61.72,42.93
  Bottom 0.254: v43.69,52.07 43.69,54.36 40.13,57.91 40.13,58.83 REF_SEL_A.3 | v61.72,42.93 60.78,41.99 56.82,41.99 v53.85,44.96
RESTESP
  Top 0.254: ESP-12.9 C21.1 64.43,10.33 65.28,11.18 69,11.18 R19.1
SCL  (via drill 0.5)
  Top 0.254: ESP-12.5 55.85,14.89 v57.66,13.08 | v71.37,16.51 71.94,15.57 72.58,15.08 PCF8523.6
  Bottom 0.254: v57.66,13.08 57.66,8.38 59.69,6.35 63.75,6.35 63.75,4.83 65.02,3.56 69.34,3.56 69.85,4.06 69.85,15.24 71.12,16.51 v71.37,16.51 71.37,24.12 P1.2
SDA  (via drill 0.5)
  Top 0.254: ESP-12.6 55.69,12.89 56.64,11.94 56.77,11.9 v56.87,11.8 | v70.87,14.22 70.87,15.24 69.85,16.26 69.85,17.21 70.51,17.86 | 70.51,17.86 70.55,17.91 73.24,17.91 PCF8523.5 | P1.1 69.44,18.93 70.51,17.86
  Bottom 0.254: v56.87,11.8 56.87,8.03 59.18,5.71 63.12,5.71 63.12,4.15 64.35,2.92 70.1,2.92 71.37,4.19 71.37,12.95 70.87,13.46 v70.87,14.22
SOURCE-NEG-A  (via drill 0.8)  (3 unrouted)
  other vias: 7.55,56.96 6.03,56.96 4.51,56.96 2.98,56.96
SOURCE-NEG-B  (via drill 0.8)  (3 unrouted)
  other vias: 7.81,38.42 6.28,38.42 4.76,38.42 3.24,38.42
SOURCE-POS-A  (via drill 0.5, 0.8)
  Top 0.152: U$3.P$1 5.59,42.93 v4.76,42.1 | U$3.P$1 5.59,42.8 v6.28,42.1 | U$3.P$1 5.78,44.13 v7.81,42.1 | U$3.P$1 5.27,44.13 v3.24,42.1
  Top 0.254: SHUNTMON-A.1 33.06,49.66 C25.1 29.72,48.86 R14.2 26.08,48.09 SCREW1.3 21.1,44.13 U$3.P$1
  Top 1.016: U$3.P$1 v5.59,47.5
  Bottom 1.016: PWR.3 arc-90 12.17,58.84 12.19,52.83 arc-90 6.86,47.5 v5.59,47.5
SOURCE-POS-B  (via drill 0.5, 0.8)  (4 unrouted)
  Top 0.254: SHUNTMON-B.1 32.73,35.69 C6.1 29.54,34.96 R1.2 28.96,34.29 27.43,34.29 27.43,27.76 SCREW2.3 20.83,25.59 U$1.P$1
  Top 1.016: U$1.P$1 v5.59,28.96
  Bottom 1.016: PWR.1 arc90 1.65,58.42 1.65,30.73 arc90 3.43,28.96 v5.59,28.96
  other vias: 8.06,23.56 6.54,23.56 5.01,23.56 3.49,23.56
VSENSEA
  Top 0.254: 28.96,44.96 R15.2 28.96,45.72 | R14.1 28.96,45.72 | MCP3208.2 69.03,53.14 68.33,53.85 43.18,53.85 41.91,52.58 41.91,48.01 40.64,46.74 34.04,46.74 33.02,45.72 28.96,45.72
VSENSEB
  Top 0.254: MCP3208.4 71.82,50.61 67.98,50.61 62.71,45.34 57.69,45.34 44.74,32.38 36.96,32.38 36.42,31.84 28.96,31.84 28.96,31.82 | 28.96,31.82 R1.1 | 28.96,31.82 R2.2
(copper drawn outside any net)
  shapes: Top area x4

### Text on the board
tPlace: VSENSE-A | VSENSE-B | MicroSD
bPlace: emonDC | wireless energy monitoring node | Technology that helps us live within ecological limits | Designed in North Wales UK by Megni | Designed in | OpenEnergyMonitor.org | North Wales | Made in UK | Node: | Open-Hardware | Format MicroSD / card to FAT32. / Place blank 'datalog.txt' / file there. | Lead free PCB - RoHS components
tNames: I1 | 470uF | 100uF | 16V | 80V | 330uH | A | B | USB_PWR | - | UNI | BI | D1 | LOAD | LMP8481 | A | GND | SOURCE | UNI | BI | + | - | LMP8481 | adc channels / 6 & 7 | LOAD | disconnect module / before FTDI flash | B | GND | LCD | SOURCE | BOOT- / LOADER / MODE | I2C | + | J1 | TX / RX | RF to ESP / (dis)connect | CRYSTAL 8x3.8mm / 32KHz
tSilk: 4.7V | 5.0V | 4.7V | RFM69Pi / RF MODULE | GND | 5V | Tx | Rx | RST | GND | emonDCduo | Wireless Energy / Monitoring Node | v1.2 Dec 2017 by DB
_tsilk: Designed in | North Wales | Made in UK
_bsilk: SMT V0.6 rev3 | emonTx | wireless energy monitoring node | SMT V0.6 rev3 | emonTx | SMT V0.6 rev3 | emonTx | Technology that helps us live within ecological limits | wireless energy monitoring node | wireless energy monitoring node | Designed in North Wales UK by Glyn Hudson & Trystan Lea | Technology that helps us live within ecological limits | Technology that helps us live within ecological limits | Designed in North Wales UK by Glyn Hudson & Trystan Lea | 165mm ant | 433Mhz | Designed in North Wales UK by Glyn Hudson & Trystan Lea | 165mm ant | 165mm ant | 433Mhz | 433Mhz | 868Mhz | 82mm ant | 82mm ant | 82mm ant | 868Mhz | 868Mhz | 78mm ant | 915Mhz | 78mm ant | 915Mhz | 78mm ant | 915Mhz | 165mm ant | 433Mhz | 82mm ant | 868Mhz | 78mm ant | 915Mhz

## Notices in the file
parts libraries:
SparkFun-Connectors: Licensing: CC v3.0 Share-Alike You are welcome to use this library for commercial purposes.
SparkFun-Aesthetics: Licensing: Creative Commons ShareAlike 4.0 International - https://creativecommons.org/licenses/by-sa/4.0
jst-ph: Copyright (C) 2016, Bob Starr
